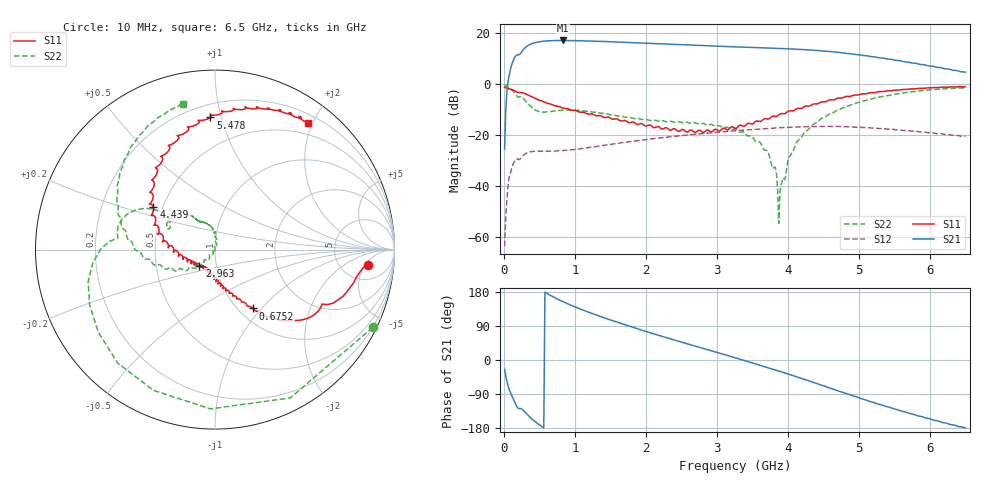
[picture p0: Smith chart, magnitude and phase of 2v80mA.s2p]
!Agilent Technologies,N5230A,MY45000233,A.04.83
!Agilent N5230A: A.04.83
!Date: Friday, August 18, 2006 03:10:04
!Correction: S11(Full 2 Port SOLT,1,2) S21(Full 2 Port SOLT,1,2) S12(Full 2 Port SOLT,1,2) S22(Full 2 Port SOLT,1,2)
!S2P File: Measurements: S11, S21, S12, S22:
# Hz S  dB  R 50
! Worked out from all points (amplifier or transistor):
!   401 points, 10 MHz to 6.5 GHz, reference 50 ohm
!   highest |S21| = 16.9 dB at 837.5 MHz (marker M1)
!   |S21| within 3 dB of that: 293.3 MHz to 3.758 GHz (3.465 GHz wide, 171 % of centre)
!   unconditionally stable (mu >= 1): start of sweep to end of sweep
!   at 1.081 GHz: K = 1.29, MAG = 17.9 dB, |S12| = -25.4 dB
!   at 3.255 GHz: K = 1.06, MAG = 14.9 dB, |S12| = -18.4 dB
!   at 6.5 GHz: K = 1.02, MAG = 11.6 dB, |S12| = -20.6 dB
!   S11 on the Smith chart (normalised r, x): 10 MHz: 9, -6; 675.2 MHz: 1.16, -0.90; 2.963 GHz: 0.83, -0.15; 4.439 GHz: 0.44, +0.26; 5.478 GHz: 0.29, +0.92; 6.5 GHz: 0.32, +1.93
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1e7  -1.32 -5.9  -25.55 -24.9  -63.55 -61.5  -0.18 -26.3
7.49e7  -2.00 -13.4  3.43 -77.9  -36.40 125.6  -1.59 -130.6
1.398e8  -2.60 -22.1  9.63 -105.7  -30.82 86.3  -3.28 -173.7
3.0205e8  -3.93 -37.4  14.15 -138.4  -27.39 49.2  -6.58 150.9
4.643e8  -6.02 -49.4  16.23 -166.3  -26.39 26.6  -10.63 148.8
6.75225e8  -8.16 -57.1  16.83 168.5  -26.37 16.0  -10.83 156.0
8.37475e8  -9.60 -61.9  16.92 153.4  -26.17 12.4  -10.32 152.1
1.097075e9  -11.15 -69.1  16.80 132.9  -25.37 8.6  -10.51 141.0
1.583825e9  -13.72 -81.3  16.31 100.4  -23.37 -1.5  -12.54 125.5
2.18415e9  -16.90 -97.5  15.59 64.9  -21.25 -20.6  -14.64 120.6
2.589775e9  -18.82 -115.8  15.12 42.3  -20.04 -35.1  -15.12 116.3
2.96295e9  -18.06 -134.3  14.69 21.9  -19.10 -49.7  -16.47 106.3
3.255e9  -17.43 -144.0  14.41 6.1  -18.42 -61.4  -17.76 101.0
3.7093e9  -13.83 -170.6  13.97 -19.5  -17.52 -81.3  -26.26 90.5
3.887775e9  -11.92 174.9  13.76 -30.1  -17.23 -89.9  -42.32 -101.7
4.0338e9  -10.58 171.7  13.59 -38.8  -17.03 -96.8  -28.04 -133.5
4.342075e9  -8.17 150.9  13.11 -58.1  -16.75 -112.7  -16.29 -136.4
4.439425e9  -7.59 145.2  12.93 -64.3  -16.70 -117.9  -14.37 -143.2
4.8775e9  -4.95 122.6  11.76 -92.0  -16.81 -140.8  -8.44 -172.0
5.42915e9  -2.80 96.7  9.59 -124.7  -17.77 -167.8  -4.48 154.8
5.477825e9  -2.65 92.0  9.39 -128.1  -17.86 -171.0  -4.26 153.3
6.5e9  -1.15 53.7  4.50 -179.7  -20.57 146.1  -1.59 102.4
